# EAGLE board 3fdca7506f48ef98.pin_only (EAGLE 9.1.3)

Size 25.4 x 25.4 mm. Coordinates in mm from the lower left corner, seen from the top.
Outline: 0,0 0,25.4 25.4,25.4 25.4,0 0,0
Copper layers (1*16): Top 0.035mm / dielectric 1.5mm / Bottom 0.035mm
Design rules "SparkFun-2-layer-FAB-LIMIT": minimum track width 4mil, minimum drill 6mil, track to track 4mil, track to pad 4mil, pad to pad 4mil, via to via 4mil, smd to smd 4mil, copper to edge 4mil, drill to drill 4mil, minimum pad ring 5mil, minimum via ring 5mil, stop-mask expansion 4mil, vias tented up to drill 25mil, thermal gap 10mil

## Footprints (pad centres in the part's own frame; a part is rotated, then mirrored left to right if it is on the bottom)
0603 = smd 1.1 x 1: 1 -0.85,0; 2 0.85,0
LED-0603 = smd 1 x 1: A -0.877,0; C 0.877,0
FIDUCIAL-1X2 = smd 1 x 1: 1 0,0
STAND-OFF = hole 3.302: 0,0
JST04_1MM_RA = smd 0.6 x 1.35: 1 -1.5,0; 2 -0.5,0; 3 0.5,0; 4 1.5,0 | smd 1.2 x 2: NC1 2.8,-3.675; NC2 -2.8,-3.675
1X06_NO_SILK = drill 1.016 pad 1.88: 1 0,0; 2 2.54,0; 3 5.08,0; 4 7.62,0; 5 10.16,0; 6 12.7,0
SMT-JUMPER_2_NO_SILK = smd 0.635 x 1.27: 1 -0.406,0; 2 0.406,0
SMT-JUMPER_3_2-NC_TRACE_SILK = smd 0.635 x 1.27: 1 -1.016,0; 2 0,0; 3 1.016,0
SMT-JUMPER_2_NC_TRACE_SILK = smd 0.635 x 1.27: 1 -0.508,0; 2 0.508,0
SOT-416FL = smd 0.46 x 0.65: 1 -0.5,-1.1; 2 0.5,-1.1; 3 0,0.05
0402-TIGHT = smd 0.6 x 0.6: 1 -0.5,0; 2 0.5,0
PAD.03X.03 = smd 0.762 x 0.762: P$1 0,0
QFN24-3X3 = smd 0.495 x 0.25: 1 -1.552,1; 6 -1.552,-1; 13 1.552,-1; 18 1.552,1 | smd 0.6 x 0.25: 2 -1.5,0.6; 3 -1.5,0.2; 4 -1.5,-0.2; 5 -1.5,-0.6; 14 1.5,-0.6; 15 1.5,-0.2; 16 1.5,0.2; 17 1.5,0.6 | smd 0.25 x 0.495: 7 -1,-1.552; 12 1,-1.552; 19 1,1.552; 24 -1,1.552 | smd 0.25 x 0.6: 8 -0.6,-1.5; 9 -0.2,-1.5; 10 0.2,-1.5; 11 0.6,-1.5; 20 0.6,1.5; 21 0.2,1.5; 22 -0.2,1.5; 23 -0.6,1.5
SC70 = smd 0.4 x 0.75: 1 -0.65,-0.825; 2 0,-0.825; 3 0.65,-0.825; 4 0.65,0.825; 5 -0.65,0.825

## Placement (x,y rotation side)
C1  1.0uF  [0603]  17.02,12.7 270 top
C2  0.1uF  [0603]  18.67,12.7 270 top
C3  0.1uF  [0603]  15.37,12.7 270 top
C4  1.0uF  [0603]  6.6,12.7 270 top
D1  RED  [LED-0603]  8.64,8.64 180 top
FD1  FIDUCIAL1X2  [FIDUCIAL-1X2]  24.64,24.64 0 top
FD2  FIDUCIAL1X2  [FIDUCIAL-1X2]  24.64,24.64 0 bottom
FD3  FIDUCIAL1X2  [FIDUCIAL-1X2]  0.76,0.76 0 bottom
FD4  FIDUCIAL1X2  [FIDUCIAL-1X2]  0.76,0.76 0 top
FRAME2  FRAME-LEDGER  [CREATIVE_COMMONS]  not placed on the board
H1  STAND-OFF  [STAND-OFF]  2.54,2.54 0 top
H2  STAND-OFF  [STAND-OFF]  22.86,2.54 0 top
H3  STAND-OFF  [STAND-OFF]  2.54,22.86 0 top
H4  STAND-OFF  [STAND-OFF]  22.86,22.86 0 top
J1  [JST04_1MM_RA]  5.08,12.7 270 top
J2  [JST04_1MM_RA]  20.32,12.7 90 top
J3  [1X06_NO_SILK]  6.35,1.27 0 top
J4  [1X06_NO_SILK]  6.35,24.13 0 top
JP2  ADR  [SMT-JUMPER_2_NO_SILK]  18.16,8.13 270 bottom
JP3  AUX  [SMT-JUMPER_3_2-NC_TRACE_SILK]  15.75,18.16 0 bottom
JP4  I2C PU  [SMT-JUMPER_3_2-NC_TRACE_SILK]  12.19,7.11 180 bottom
JP5  LED  [SMT-JUMPER_2_NC_TRACE_SILK]  8.76,12.7 270 bottom
LOGO1  SFE_LOGO_NAME_FLAME.1_INCH  [SFE_LOGO_NAME_FLAME_.1]  20.95,12.7 90 bottom
LOGO2  OSHW-LOGOMINI  [OSHW-LOGO-MINI]  24.13,7.24 90 top
Q2  20V/0.2A/8MHz/1.2Ω/1Vth  [SOT-416FL]  19.05,7.37 180 top
Q4  20V/0.2A/8MHz/1.2Ω/1Vth  [SOT-416FL]  16.51,7.37 180 top
Q6  20V/0.2A/8MHz/1.2Ω/1Vth  [SOT-416FL]  13.97,7.37 180 top
Q8  20V/0.2A/8MHz/1.2Ω/1Vth  [SOT-416FL]  11.43,7.37 180 top
Q10  20V/0.2A/8MHz/1.2Ω/1Vth  [SOT-416FL]  13.97,18.03 0 top
Q12  20V/0.2A/8MHz/1.2Ω/1Vth  [SOT-416FL]  16.51,18.03 0 top
Q14  20V/0.2A/8MHz/1.2Ω/1Vth  [SOT-416FL]  11.43,18.03 0 top
Q16  20V/0.2A/8MHz/1.2Ω/1Vth  [SOT-416FL]  8.89,18.03 0 top
R9  220  [0603]  8.64,10.29 180 top
R10  2.2k  [0402-TIGHT]  19.05,9.53 0 top
R11  2.2k  [0402-TIGHT]  19.05,6.22 180 top
R12  2.2k  [0402-TIGHT]  16.51,9.53 0 top
R13  2.2k  [0402-TIGHT]  16.51,6.22 180 top
R14  2.2k  [0402-TIGHT]  13.97,9.53 0 top
R15  2.2k  [0402-TIGHT]  13.97,6.22 180 top
R16  2.2k  [0402-TIGHT]  11.43,9.53 0 top
R17  2.2k  [0402-TIGHT]  11.43,6.22 180 top
R18  2.2k  [0402-TIGHT]  13.97,15.88 180 top
R19  2.2k  [0402-TIGHT]  13.97,19.18 0 top
R20  2.2k  [0402-TIGHT]  16.51,15.88 180 top
R21  2.2k  [0402-TIGHT]  16.51,19.18 0 top
R22  2.2k  [0402-TIGHT]  11.43,15.88 180 top
R23  2.2k  [0402-TIGHT]  11.43,19.18 0 top
R24  2.2k  [0402-TIGHT]  8.89,15.88 180 top
R25  2.2k  [0402-TIGHT]  8.89,19.18 0 top
TP1  1.8V  [PAD.03X.03]  10.16,20.32 0 bottom
U2  9DoF IMU  [QFN24-3X3]  12.7,12.7 180 top
U3  1.8V/100mA  [SC70]  8.64,12.7 270 top
U$1  [GND4]  6.35,2.03 90 bottom
U$2  [GND4]  6.35,19.81 90 bottom
U$3  [PWR0]  6.35,6.86 90 top
U$4  [INT3]  8.89,20.57 90 bottom
U$5  [FSNC2]  11.43,19.56 90 bottom
U$6  [ACL1]  16.51,20.19 90 bottom
U$7  [ADA0]  13.97,20.07 90 bottom
U$8  [MISO13]  16.51,1.65 90 bottom
U$9  [MOSI14]  11.43,1.65 90 bottom
U$10  [SCLK15]  13.97,1.65 90 bottom
U$11  [#CS16]  19.05,1.52 90 bottom
U$12  [1V8#5V57]  8.89,1.65 90 bottom
U$13  [VIN5]  8.89,1.65 90 top
U$14  [NC17]  19.05,1.91 90 top
U$15  [CL4]  13.97,1.65 90 top
U$16  [DA2]  11.43,1.65 90 top
U$17  [AD012]  16.51,1.65 90 top
U$18  [ADA0]  13.97,20.07 90 top
U$19  [ACL1]  16.51,20.19 90 top
U$20  [FSNC2]  11.43,19.56 90 top
U$21  [INT3]  8.89,20.57 90 top
U$22  [GND4]  6.35,2.03 90 top
U$23  [ADR2]  18.16,8.64 90 bottom
U$24  [GND4]  6.35,19.81 90 top
U$25  [I2C_PU21]  12.19,7.62 90 bottom
U$26  [SPI19]  24.13,4.19 90 bottom
U$27  [AUX_PU24]  15.75,10.41 90 bottom
U$28  [SFE_LOGO_FLAME_.1]  21.59,7.11 90 top
U$29  [LED23]  8.76,7.49 90 bottom
U$30  [VIN5]  19.05,20.45 90 top
U$31  [ICM#2094820]  1.59,6.92 90 bottom
U$34  [X0]  1.85,19.96 180 top
U$35  [Y1]  5.54,16.71 180 top
U$36  [Z2]  2.11,16.71 180 top
U$37  [G5]  4.78,19.89 180 top
U$38  [A4]  5.79,19.89 180 top
U$39  [M3]  25.52,16.82 180 top
U$40  [X0]  20.04,15.22 90 top
U$41  [Y1]  25.34,19.66 180 top
U$42  [Z2]  19.69,19.79 0 top
U$43  [QWIIC_9DOF_IMU_0]  3.68,4.89 90 bottom
U$44  [VIN5]  19.05,20.45 90 bottom
U$45  [I#C1]  1.37,4.25 90 top
U$49  [M3]  6.99,15.04 180 bottom
U$50  [X0]  4.17,14.96 180 bottom
U$51  [Y1]  7.81,18.64 180 bottom
U$52  [Z2]  4.45,18.69 180 bottom
U$57  [X0]  11.25,18.77 0 bottom
U$58  [Y1]  12.37,14.68 180 bottom
U$59  [Z2]  11,14.91 0 bottom
U$60  [G5]  12.37,18.49 180 bottom
U$61  [A4]  11.35,18.49 180 bottom

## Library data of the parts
C1 C4 = SparkFun-Capacitors; PROD_ID: CAP-13930
C2 C3 = SparkFun-Capacitors; PROD_ID: CAP-08604
D1 = SparkFun-LED; PROD_ID: DIO-00819
FD1-FD4 LOGO1 LOGO2 U$28 = SparkFun-Aesthetics
FRAME2 = SparkFun-Aesthetics; DESIGNER: Owen Lyke; REV: v31
H1-H4 = SparkFun-Hardware
J1 J2 = SparkFun-Connectors; PROD_ID: CONN-13694
J3 J4 TP1 = SparkFun-Connectors
JP2-JP5 = SparkFun-Jumpers
Q2 Q4 Q6 Q8 Q10 Q12 Q14 Q16 = SparkFun-DiscreteSemi; PROD_ID: TRANS_14399
R9 = SparkFun-Resistors; PROD_ID: RES-07861
R10-R25 = SparkFun-Resistors; PROD_ID: RES-14341
U2 = SparkFun-Sensors; PROD_ID: IC-14247
U3 = SparkFun-IC-Power; PROD_ID: VREG-08428
U$1 U$2 U$4-U$14 U$17-U$22 U$24-U$27 U$29 U$30 U$44 = buzzard_labels_2
U$3 U$23 U$45 = buzzard_labels_4
U$15 U$16 U$31 U$43 = buzzard_labels
U$34-U$42 U$49-U$52 U$57-U$61 = buzzard_labels (1)

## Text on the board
Bottom: v31
tDocu: Owen Lyke

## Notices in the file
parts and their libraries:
SparkFun-Connectors: Licensing: Creative Commons ShareAlike 4.0 International - https://creativecommons.org/licenses/by-sa/4.0
SparkFun-Aesthetics: Released under the Creative Commons Attribution Share-Alike 4.0 License
SparkFun-Aesthetics: https://creativecommons.org/licenses/by-sa/4.0
